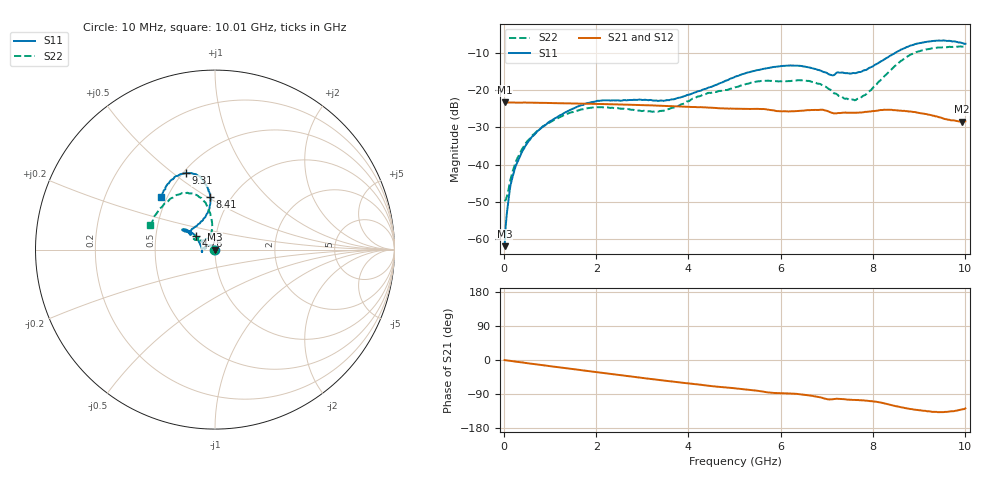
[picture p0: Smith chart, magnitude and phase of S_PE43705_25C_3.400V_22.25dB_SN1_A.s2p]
! Device ID: PE43705
! Serial: 1
! Insertion: A
! Impedance: 50 ohm
! Temp: 25C
! VDD: 3.400V
! Attenuation Step: 22.25dB
#  Hz  S  RI  R  50
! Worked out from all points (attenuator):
!   401 points, 10 MHz to 10.01 GHz, reference 50 ohm
!   highest |S21| = -23.28 dB at 10 MHz (marker M1); lowest = -28.5 dB at 9.935 GHz (marker M2)
!   lowest |S11| = -61.9 dB at 10 MHz (marker M3), VSWR 1.00, Z = 49.9 + j0.0426 ohm
!   |S11| at or under -10 dB: start of sweep to 8.485 GHz
!   |S22| runs from -49.8 to -8.3 dB; largest |S21 - S12| = 0.00097
!   S11 on the Smith chart (normalised r, x): 10 MHz: 1.00, +0.00; 4.76 GHz: 0.80, +0.12; 8.41 GHz: 0.80, +0.52; 9.31 GHz: 0.52, +0.56; 10.01 GHz: 0.46, +0.33
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1e7  -0.000685 0.000427  0.0685 -0.000281  0.0686 -0.000278  -0.00322 0.000409
1.1e8  -0.000454 0.00399  0.0682 -0.00227  0.0682 -0.00223  -0.00267 0.00452
1.85e8  -0.00119 0.00684  0.0681 -0.00374  0.0681 -0.00372  -0.00305 0.0076
4.35e8  -0.00602 0.0155  0.0676 -0.00864  0.0673 -0.00849  -0.00707 0.0165
8.6e8  -0.0244 0.0226  0.0655 -0.0164  0.0654 -0.0163  -0.0221 0.0244
1.685e9  -0.062 0.00981  0.0588 -0.0299  0.0588 -0.0299  -0.0526 0.0169
2.16e9  -0.0727 -0.00487  0.0537 -0.0367  0.0537 -0.0367  -0.0581 0.00721
3.36e9  -0.0717 -0.00399  0.0375 -0.0492  0.0374 -0.0492  -0.0502 0.0131
4.76e9  -0.1062 0.0738  0.0177 -0.0541  0.0178 -0.0542  -0.0812 0.0583
5.01e9  -0.1218 0.089  0.0147 -0.0543  0.0147 -0.0543  -0.0886 0.0635
5.535e9  -0.1533 0.1067  0.00768 -0.0553  0.0078 -0.0554  -0.1082 0.0741
5.985e9  -0.1766 0.1134  0.00253 -0.052  0.00257 -0.0519  -0.11 0.0711
6.685e9  -0.1684 0.1009  -0.00429 -0.0539  -0.00453 -0.0538  -0.1148 0.0583
7.11e9  -0.1332 0.0863  -0.0118 -0.0483  -0.0116 -0.048  -0.0818 0.0528
7.61e9  -0.0893 0.1433  -0.0132 -0.0479  -0.0131 -0.0477  -0.0376 0.0626
7.885e9  -0.0521 0.1841  -0.0155 -0.0489  -0.0155 -0.0489  -0.0227 0.0899
8.36e9  -0.0249 0.2837  -0.0253 -0.0483  -0.0252 -0.0481  -0.0211 0.1784
8.41e9  -0.0278 0.2953  -0.0265 -0.0476  -0.0262 -0.0476  -0.0244 0.189
8.86e9  -0.0767 0.3957  -0.0327 -0.0393  -0.0326 -0.0391  -0.0884 0.2931
9.31e9  -0.1628 0.4266  -0.033 -0.0311  -0.033 -0.0314  -0.1898 0.3118
9.935e9  -0.2917 0.3148  -0.0245 -0.0287  -0.0248 -0.029  -0.3451 0.1659
1.001e10  -0.2995 0.2922  -0.0233 -0.0302  -0.0239 -0.03  -0.3607 0.1367
